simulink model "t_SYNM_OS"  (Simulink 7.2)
settings: Solver=ode3  SolverMode=SingleTasking  StartTime=0.0  StopTime=1.5  FixedStep=5e-6  RelTol=1e-6  AbsTol=1e-6
libraries: simulink x1

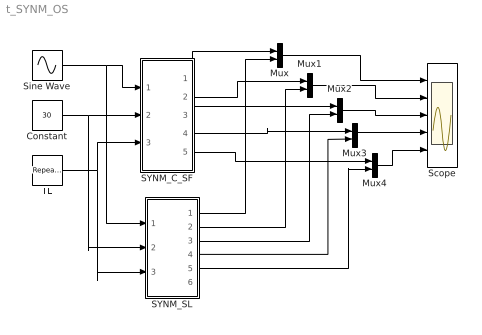
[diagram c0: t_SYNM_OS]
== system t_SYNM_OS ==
  Constant : Constant  Value=30
  Mux{,1..4} (5 alike) : Mux  Inputs=2
  SYNM_C_SF : Subsystem  mask(Syn. MOTOR C-S-Function Block){rs=0.1, Lls=0.79e-3, rk=0.17, Llkq=0.91e-3, Llkd=0.29e-3, Lmq=2e-3, Lmd=4.1e-3, rf=.16, Llf=0.38e-3, P=4, J=.2, D=0.05}
      mask prompts: rs "Stator Resistance"; Lls "Stator Leakage Inductance"; rk "Damper Winding Resistance"; Llkq "Damper Q-Axis Leakage Inductance"; Llkd "Damper D-Axis Leakage Inductance"; Lmq "Q-Axis Magnetising Inductance"; Lmd "D-Axis Magnetising Inductance"; rf "Field  Winding Resistance"; Llf "Field Winding Leakage Inductance"; P "Number of Poles"; J "Moment of Inertia"; D "Damping Coefficient"
      mask help: Open source Syn. MOTOR modeled as Simulink C-S-Function Block Input Vector u: u[0,1,2]= Three phase stator Voltages u[3] = Field DC-Voltages u[4] = Load Torque Output Vector y: y[0,1,2]= Three phase stator Currents y[3]= Te y[4]= Ang. Velocity W y[5]= Field DC-Current Parameter Vector p: p[0]= Stator Resistance rs p[1]= Stator Leakage Inductance Lls p[2]= Damper Winding Resistance rk p[3]= Damper Q-Axis Leakage Inductance Llkq p[4]= Damper D-Axis Leakage Inductance Llkd p[5]= Q-Axis Magnetising Inductance Lmq p[6]= D-Axis Magnetising Inductance Lmd p[7]= Field Winding Resistance rf p[8]= Field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
  SYNM_SL : Subsystem  mask(Syn. MOTOR Simulink Blocks){rs=0.1, Lls=0.79e-3, rk=0.17, Llkq=0.91e-3, Llkd=0.29e-3, Lmq=2e-3, Lmd=4.1e-3, rf=.16, Llf=0.38e-3, P=4, J=.2, D=0.05, omm0=0}
      mask prompts: rs "Stator Resistance"; Lls "Stator  Leakage Inductance"; rk "Damper Winding Resistance"; Llkq "Damper Q-Axis Leakage Inductance"; Llkd "Damper D-Axis Leakage Inductance"; Lmq "Q-Axis Magnetising Inductance"; Lmd "D-Axis Magnetising Inductance"; rf "Field  Winding Resistance"; Llf "Field Winding Leakage Inductance"; P "Number of Poles"; J "Moment of Inertia"; D "Damping Coefficient"; omm0 "initial ang. speed"
      mask help: Open source Syn. MOTOR modeled in Simulink Blocks Input Vector u: u[0,1,2]= Three phase stator Voltages u[3] = Field DC-Voltages u[4] = Load Torque Output Vector y: y[0,1,2]= Three phase stator Currents y[3]= Te y[4]= Ang. Velocity W y[5]= Field DC-Current Parameter Vector p: p[0]= Stator Resistance rs p[1]= Stator Leakage Inductance Lls p[2]= Damper Winding Resistance rk p[3]= Damper Q-Axis Leakage Inductance Llkq p[4]= Damper D-Axis Leakage Inductance Llkd p[5]= Q-Axis Magnetising Inductance Lmq p[6]= D-Axis Magnetising Inductance Lmd p[7]= Field Winding Resistance rf p[8]= Field Winding Lea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
  Scope : Scope  NumInputPorts=5
  Sine Wave : Sin  Amplitude=188  Frequency=377  Phase="[pi/2  -2*pi/3+pi/2   -4*pi/3+pi/2]"  SampleTime=0
  TL : simulink/Sources/Repeating Sequence  SystemSampleTime=-1  rep_seq_t="[0      0.8     0.801      1.2     1.201      2 ]"  rep_seq_y="[0       0        200        200     -200   -200]"
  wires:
  Sine Wave/1 -> SYNM_SL/1(Vabc), SYNM_C_SF/1(Vabc)
  TL/1 -> SYNM_SL/3(Tl), SYNM_C_SF/3(TL)
  Constant/1 -> SYNM_SL/2(Vfd), SYNM_C_SF/2(Vdf)
  SYNM_C_SF/1(iA) -> Mux/1
  SYNM_C_SF/2(iB) -> Mux1/1
  SYNM_C_SF/3(iC) -> Mux2/1
  SYNM_C_SF/4(TE) -> Mux3/1
  SYNM_C_SF/5(W) -> Mux4/1
  SYNM_SL/1(ia) -> Mux/2
  SYNM_SL/2(ib) -> Mux1/2
  SYNM_SL/3(ic) -> Mux2/2
  SYNM_SL/4(Te) -> Mux3/2
  SYNM_SL/5(w) -> Mux4/2
  Mux/1 -> Scope/1
  Mux1/1 -> Scope/2
  Mux2/1 -> Scope/3
  Mux3/1 -> Scope/4
  Mux4/1 -> Scope/5

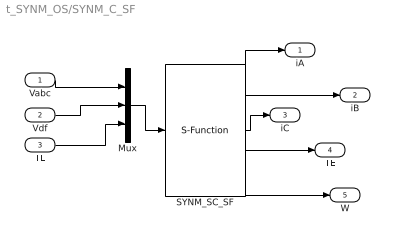
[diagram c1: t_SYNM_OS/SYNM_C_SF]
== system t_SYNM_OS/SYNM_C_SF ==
  Vabc : Inport  OutDataType=sfix(16)  OutScaling=2^0
  Vdf : Inport  Port=2  OutDataType=sfix(16)  OutScaling=2^0
  TL : Inport  Port=3  OutDataType=sfix(16)  OutScaling=2^0
  Mux : Mux  Inputs="[3 1   1]"
  SYNM_SC_SF : S-Function  FunctionName=s_Synm_OS  Parameters="[rs Lls rk Llkq  Llkd Lmq Lmd rf  Llf  P J D]"  EnableBusSupport=off
  iA : Outport  OutDataType=sfix(16)  OutScaling=2^0
  iB : Outport  Port=2  OutDataType=sfix(16)  OutScaling=2^0
  iC : Outport  Port=3  OutDataType=sfix(16)  OutScaling=2^0
  TE : Outport  Port=4  OutDataType=sfix(16)  OutScaling=2^0
  W : Outport  Port=5  OutDataType=sfix(16)  OutScaling=2^0
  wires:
  Mux/1 -> SYNM_SC_SF/1
  Vabc/1 -> Mux/1
  TL/1 -> Mux/3
  SYNM_SC_SF/2 -> iB/1
  SYNM_SC_SF/3 -> iC/1
  SYNM_SC_SF/1 -> iA/1
  SYNM_SC_SF/4 -> TE/1
  SYNM_SC_SF/5 -> W/1
  Vdf/1 -> Mux/2

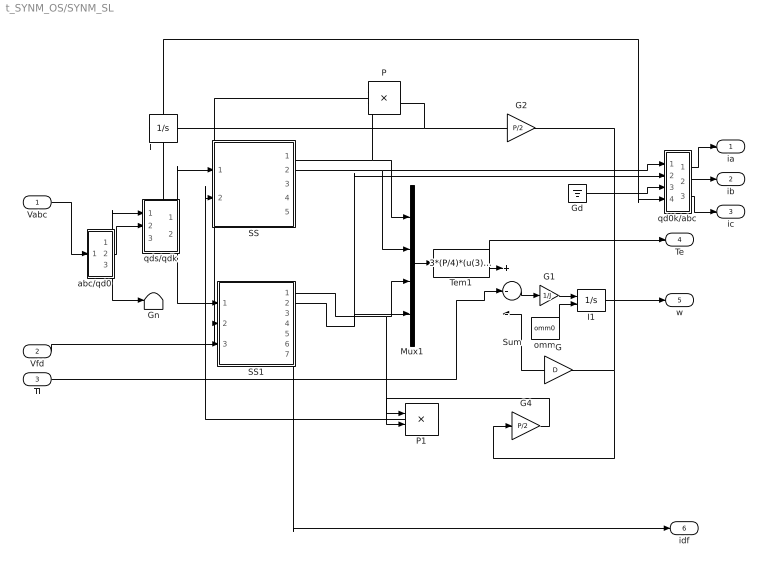
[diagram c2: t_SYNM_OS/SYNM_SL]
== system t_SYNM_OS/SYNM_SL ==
  Vabc : Inport
  Vfd : Inport  Port=2
  Tl : Inport  Port=3
  G : Gain  Gain=D
  G1 : Gain  Gain=1/J
  G2 : Gain  Gain=P/2
  G4 : Gain  Gain=P/2
  Gd : Ground
  Gn : Terminator
  I : Integrator
  I1 : Integrator  InitialConditionSource=external
  Mux1 : Mux
  P : Product
  P1 : Product
  SS : Subsystem
  SS1 : Subsystem
  Sum : Sum  Inputs=+--
  Tem1 : Fcn  Expr=3*(P/4)*(u(3)*u(2)-u(1)*u(4))
  abc/qd0 : Subsystem
  omm : Constant  Value=omm0
  qd0k/abc : Subsystem
  qds/qdk : Subsystem
  ia : Outport
  ib : Outport  Port=2
  ic : Outport  Port=3
  Te : Outport  Port=4
  w : Outport  Port=5
  idf : Outport  Port=6
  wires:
  Gd/1 -> qd0k/abc/3(0k)
  qd0k/abc/2(b) -> ib/1
  qd0k/abc/1(a) -> ia/1
  P/1 -> SS1/2(wr*psiqs)
  G2/1 -> P/2, I/1
  Vabc/1 -> abc/qd0/1(abc)
  abc/qd0/2(d) -> qds/qdk/2(ds)
  Vfd/1 -> SS1/3(udf)
  qds/qdk/2(dk) -> SS1/1(uds)
  qds/qdk/1(qk) -> SS/1(uqs)
  SS1/7(idf) -> idf/1
  SS/1(psiqs) -> Mux1/1, P/1
  abc/qd0/3(0) -> Gn/1
  abc/qd0/1(q) -> qds/qdk/1(qs)
  Mux1/1 -> Tem1/1
  Sum/1 -> G1/1
  G4/1 -> P1/2
  P1/1 -> SS/2(wr*psids)
  I1/1 -> G2/1, w/1, G4/1, G/1
  G/1 -> Sum/3
  SS/2(iqs) -> Mux1/2, qd0k/abc/1(qk)
  Tem1/1 -> Sum/1, Te/1
  Tl/1 -> Sum/2
  SS1/2(ids) -> Mux1/4, qd0k/abc/2(dk)
  SS1/1(psids) -> P1/1, Mux1/3
  I/1 -> qds/qdk/3(th), qd0k/abc/4(th)
  qd0k/abc/3(c) -> ic/1
  G1/1 -> I1/1
  omm/1 -> I1/2

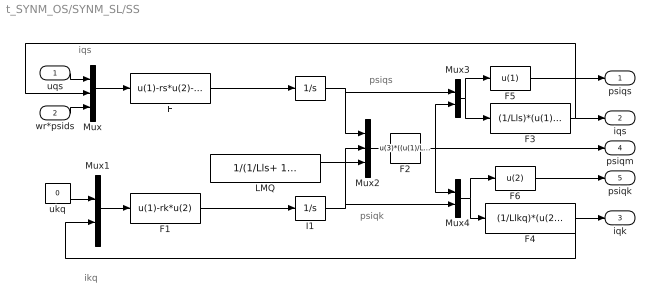
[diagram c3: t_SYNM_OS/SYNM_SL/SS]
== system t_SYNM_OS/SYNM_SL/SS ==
  note: psiqs
  note: psiqk
  note: ikq
  note: iqs
  uqs : Inport
  wr*psids : Inport  Port=2
  F : Fcn  Expr=u(1)-rs*u(2)-u(3)
  F1 : Fcn  Expr=u(1)-rk*u(2)
  F2 : Fcn  Expr=u(3)*((u(1)/Lls)+(u(2)/Llkq))
  F3 : Fcn  Expr=(1/Lls)*(u(1)-u(2))
  F4 : Fcn  Expr=(1/Llkq)*(u(2)-u(1))
  F5 : Fcn  Expr=u(1)
  F6 : Fcn  Expr=u(2)
  I : Integrator
  I1 : Integrator
  LMQ : Constant  Value=1/(1/Lls+ 1/Llkq+ 1/Lmq)
  Mux : Mux  Inputs=3
  Mux1 : Mux  Inputs=2
  Mux2 : Mux  Inputs=3
  Mux3 : Mux  Inputs=2
  Mux4 : Mux  Inputs=2
  ukq : Constant  Value=0
  psiqs : Outport
  iqs : Outport  Port=2
  iqk : Outport  Port=3
  psiqm : Outport  Port=4
  psiqk : Outport  Port=5
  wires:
  F6/1 -> psiqk/1
  F2/1 -> psiqm/1, Mux3/2, Mux4/1
  Mux3/1 -> F3/1, F5/1
  F5/1 -> psiqs/1
  Mux4/1 -> F4/1, F6/1
  F3/1 -> iqs/1, Mux/2
  F4/1 -> iqk/1, Mux1/2
  wr*psids/1 -> Mux/3
  Mux/1 -> F/1
  F/1 -> I/1
  Mux1/1 -> F1/1
  Mux2/1 -> F2/1
  I/1 -> Mux2/1, Mux3/1
  I1/1 -> Mux4/2, Mux2/2
  uqs/1 -> Mux/1
  F1/1 -> I1/1
  ukq/1 -> Mux1/1
  LMQ/1 -> Mux2/3

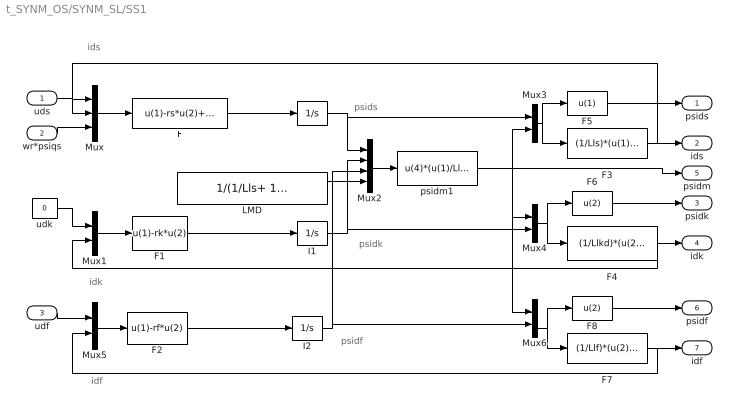
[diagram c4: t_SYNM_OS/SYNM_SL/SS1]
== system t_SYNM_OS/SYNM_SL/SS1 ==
  note: idf
  note: psidf
  note: psids
  note: psidk
  note: ids
  note: idk
  uds : Inport
  wr*psiqs : Inport  Port=2
  udf : Inport  Port=3
  F : Fcn  Expr=u(1)-rs*u(2)+u(3)
  F1 : Fcn  Expr=u(1)-rk*u(2)
  F2 : Fcn  Expr=u(1)-rf*u(2)
  F3 : Fcn  Expr=(1/Lls)*(u(1)-u(2))
  F4 : Fcn  Expr=(1/Llkd)*(u(2)-u(1))
  F5 : Fcn  Expr=u(1)
  F6 : Fcn  Expr=u(2)
  F7 : Fcn  Expr=(1/Llf)*(u(2)-u(1))
  F8 : Fcn  Expr=u(2)
  I : Integrator
  I1 : Integrator
  I2 : Integrator
  LMD : Constant  Value=1/(1/Lls+ 1/Llf+ 1/Llkd+ 1/Lmd)
  Mux : Mux  Inputs=3
  Mux{1,3..6} (5 alike) : Mux  Inputs=2
  Mux2 : Mux
  psidm1 : Fcn  Expr=u(4)*(u(1)/Lls+u(2)/Llkd+u(3)/Llf)
  udk : Constant  Value=0
  psids : Outport
  ids : Outport  Port=2
  psidk : Outport  Port=3
  idk : Outport  Port=4
  psidm : Outport  Port=5
  psidf : Outport  Port=6
  idf : Outport  Port=7
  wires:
  LMD/1 -> Mux2/4
  I2/1 -> Mux2/3, Mux6/2
  F8/1 -> psidf/1
  Mux6/1 -> F7/1, F8/1
  F7/1 -> Mux5/2, idf/1
  F2/1 -> I2/1
  Mux5/1 -> F2/1
  udf/1 -> Mux5/1
  wr*psiqs/1 -> Mux/3
  F6/1 -> psidk/1
  Mux4/1 -> F6/1, F4/1
  F5/1 -> psids/1
  Mux3/1 -> F5/1, F3/1
  uds/1 -> Mux/1
  I1/1 -> Mux4/2, Mux2/2
  I/1 -> Mux3/1, Mux2/1
  Mux2/1 -> psidm1/1
  Mux1/1 -> F1/1
  F/1 -> I/1
  Mux/1 -> F/1
  F1/1 -> I1/1
  udk/1 -> Mux1/1
  F3/1 -> ids/1, Mux/2
  F4/1 -> idk/1, Mux1/2
  psidm1/1 -> Mux6/1, Mux4/1, Mux3/2, psidm/1

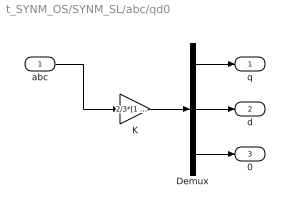
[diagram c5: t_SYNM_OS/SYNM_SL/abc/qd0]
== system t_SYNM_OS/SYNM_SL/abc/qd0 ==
  abc : Inport
  Demux : Demux  Outputs=3
  K : Gain  Gain="2/3*[1   -.5   -.5;  0   -sqrt(3)/2   sqrt(3)/2;  .5    .5    .5]"  Multiplication=Matrix(K*u)
  q : Outport
  d : Outport  Port=2
  0 : Outport  Port=3
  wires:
  Demux/3 -> 0/1
  Demux/2 -> d/1
  Demux/1 -> q/1
  abc/1 -> K/1
  K/1 -> Demux/1

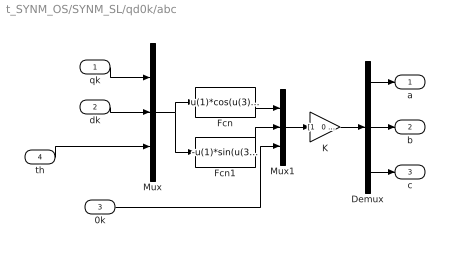
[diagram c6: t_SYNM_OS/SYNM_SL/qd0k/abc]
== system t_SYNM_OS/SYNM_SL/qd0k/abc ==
  qk : Inport
  dk : Inport  Port=2
  0k : Inport  Port=3
  th : Inport  Port=4
  Demux : Demux  Outputs=3
  Fcn : Fcn  Expr=u(1)*cos(u(3)) + u(2)*sin(u(3))
  Fcn1 : Fcn  Expr=-u(1)*sin(u(3)) + u(2)*cos(u(3))
  K : Gain  Gain="[1   0  1 ;  -.5   -sqrt(3)/2    1 ;  -.5    sqrt(3)/2    1]"  Multiplication=Matrix(K*u)
  Mux : Mux  Inputs=3
  Mux1 : Mux  Inputs=3
  a : Outport
  b : Outport  Port=2
  c : Outport  Port=3
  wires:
  qk/1 -> Mux/1
  dk/1 -> Mux/2
  Mux/1 -> Fcn/1, Fcn1/1
  K/1 -> Demux/1
  Mux1/1 -> K/1
  Fcn/1 -> Mux1/1
  Fcn1/1 -> Mux1/2
  Demux/1 -> a/1
  Demux/2 -> b/1
  Demux/3 -> c/1
  th/1 -> Mux/3
  0k/1 -> Mux1/3

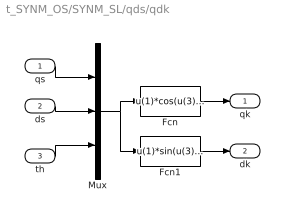
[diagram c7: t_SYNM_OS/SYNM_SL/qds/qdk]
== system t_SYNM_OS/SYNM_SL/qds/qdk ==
  qs : Inport
  ds : Inport  Port=2
  th : Inport  Port=3
  Fcn : Fcn  Expr=u(1)*cos(u(3)) - u(2)*sin(u(3))
  Fcn1 : Fcn  Expr=u(1)*sin(u(3)) + u(2)*cos(u(3))
  Mux : Mux  Inputs=3
  qk : Outport
  dk : Outport  Port=2
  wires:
  Fcn1/1 -> dk/1
  Fcn/1 -> qk/1
  Mux/1 -> Fcn1/1, Fcn/1
  th/1 -> Mux/3
  ds/1 -> Mux/2
  qs/1 -> Mux/1
